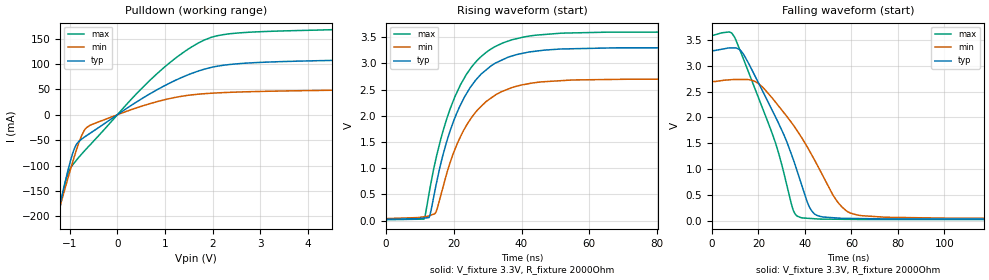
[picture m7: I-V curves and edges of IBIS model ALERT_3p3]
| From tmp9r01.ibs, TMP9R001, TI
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|   Model
[Model]   ALERT_3p3
Model_type   Open_drain
Polarity   Non-Inverting
Vmeas = 1.65
Vref = 3.3
Cref = 1pF
Rref = 2000
|   typ   min   max
C_comp   1.523pF   1.378pF   1.601pF
[Voltage Range]   3.3   2.7   3.6
[Temperature Range]   25   125   -40
[Pullup Reference]   3.3   2.7   3.6
[Pulldown Reference]   0   0   0
[Power Clamp Reference]   3.3   2.7   3.6
[GND Clamp Reference]   0   0   0
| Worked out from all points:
|   slope of the pulldown table from 0 to 0.495 V, typ, clamps not added: 16.2 ohm
|   falling waveform, V_fixture 3.3V, R_fixture 2000Ohm: 20-80 % time 18.4ns typ, 21.6ns min, 16.3ns max; typ from 3.3 V to 0.025 V
|   rising waveform, V_fixture 3.3V, R_fixture 2000Ohm: 20-80 % time 11.3ns typ, 11.3ns min, 11.4ns max; typ from 0.025 V to 3.3 V
[Pulldown]
|   Voltage   I(typ)   I(min)   I(max)
-3.3V     -1.115A    -955.3mA   -1.287A
-1.369V   -246mA     -238.4mA   -263.3mA
-1.261V   -199.9mA   -200.5mA   -209.5mA
-1.122V   -142.9mA   -153.3mA   -145.8mA
-1.033V   -108.4mA   -123.6mA   -114.6mA
-864.6mV  -59.23mA   -70.95mA   -90.13mA
-755.7mV  -48.36mA   -42.33mA   -78.07mA
-646.8mV  -41.17mA   -25.32mA   -66.84mA
848.1mV   50.03mA    26.17mA    82.24mA
1.818V    89.56mA    41.4mA     146.9mA
2.788V    102.1mA    45.41mA    162.6mA
6.6V      111.2mA    51.14mA    172.8mA
[Ramp]
R_load = 2000
|   typ   min   max
dV/dt_r   1.96491/1.12793e-08   1.59755/1.13041e-08   2.15001/1.14327e-08
dV/dt_f   1.9649/1.83583e-08   1.59748/2.14747e-08   2.15001/1.62602e-08
[Falling Waveform]
V_fixture = 3.3V
V_fixture_min = 2.7V
V_fixture_max = 3.6V
R_fixture = 2000Ohm
C_fixture = 0F
|   Time   V(typ)   V(min)   V(max)
0s        3.3V       2.7V       3.6V
9.739ns   3.349V     2.737V     3.554V
21.3ns    2.556V     2.608V     2.232V
27.83ns   1.965V     2.269V     1.434V
34.82ns   1.207V     1.863V     218.5mV
38.26ns   735.8mV    1.631V     57.32mV
44.28ns   122mV      1.16V      34.29mV
54.88ns   45.93mV    315.2mV    24.8mV
64.42ns   37.94mV    94.22mV    20.7mV
300ns     25.17mV    37.54mV    16.66mV
[Rising Waveform]
V_fixture = 3.3V
V_fixture_min = 2.7V
V_fixture_max = 3.6V
R_fixture = 2000Ohm
C_fixture = 0F
|   Time   V(typ)   V(min)   V(max)
0s        25.14mV    37.41mV    16.65mV
11.19ns   47.34mV    72.71mV    26.9mV
12.66ns   56.56mV    89.04mV    505mV
14.68ns   653.2mV    155.8mV    1.166V
16.81ns   1.256V     637.4mV    1.709V
19.65ns   1.847V     1.246V     2.254V
23.14ns   2.358V     1.749V     2.725V
31.06ns   2.956V     2.341V     3.277V
40.61ns   3.196V     2.595V     3.503V
300ns     3.3V       2.7V       3.6V
